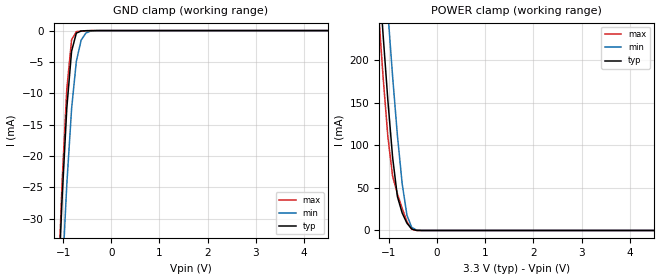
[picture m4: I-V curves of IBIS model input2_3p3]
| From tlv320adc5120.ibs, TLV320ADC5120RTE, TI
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|   input2_3p3 Model
[Model]   input2_3p3
Model_type   Input
Vinl = 0.8
Vinh = 2
|   typ   min   max
C_comp   4.663pF   4.5044pF   4.717pF
| Where Nom  PVT is Nominal Process, 3.3V, 27C
|   Fast PVT is Strong Process,  3.6V, -40C
|   Slow PVT is Weak Process,   3.0V, 150C
[Voltage Range]   3.3   3   3.6
|Junction Temperature
[Temperature Range]   27   150   -40
[Power Clamp Reference]   3.3   3   3.6
[GND Clamp Reference]   0   0   0
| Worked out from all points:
|   GND clamp passes 1 mA (typ) near -0.75 V on its own axis
|   POWER clamp passes 1 mA (typ) near -0.48 V on its own axis
[GND Clamp]
|   Voltage   I(typ)   I(min)   I(max)
-3.3V     -587.5mA   -559.8mA   -668.7mA
-1.122V   -44.97mA   -57.14mA   -44.41mA
-1.023V   -26.94mA   -39.8mA    -24.33mA
-924mV    -12.32mA   -24.5mA    -9.315mA
-825mV    -3.288mA   -12.47mA   -1.467mA
-726mV    -402.2uA   -4.899mA   -169uA
-627mV    -73.41uA   -1.536mA   -63.78uA
-528mV    -22.58uA   -387.1uA   -22.9uA
-429mV    -9.621uA   -74.49uA   -11.25uA
6.6V      0A         0A         0A
[POWER Clamp]
|   Voltage   I(typ)   I(min)   I(max)
-3.3V     2.18A      2.271A     2.137A
-1.221V   312mA      419.1mA    260.3mA
-1.122V   230.1mA    336.6mA    180.4mA
-1.023V   152.9mA    256.6mA    110.2mA
-924mV    85.72mA    180.7mA    63.62mA
-825mV    39.91mA    111.8mA    43.21mA
-726mV    20.58mA    55.13mA    26.23mA
-627mV    8.573mA    18mA       10.45mA
-528mV    1.742mA    3.661mA    1.568mA
-429mV    116uA      559.4uA    40.33uA
-231mV    15.04nA    7.154uA    182.3nA
6.6V      0A         0A         0A
